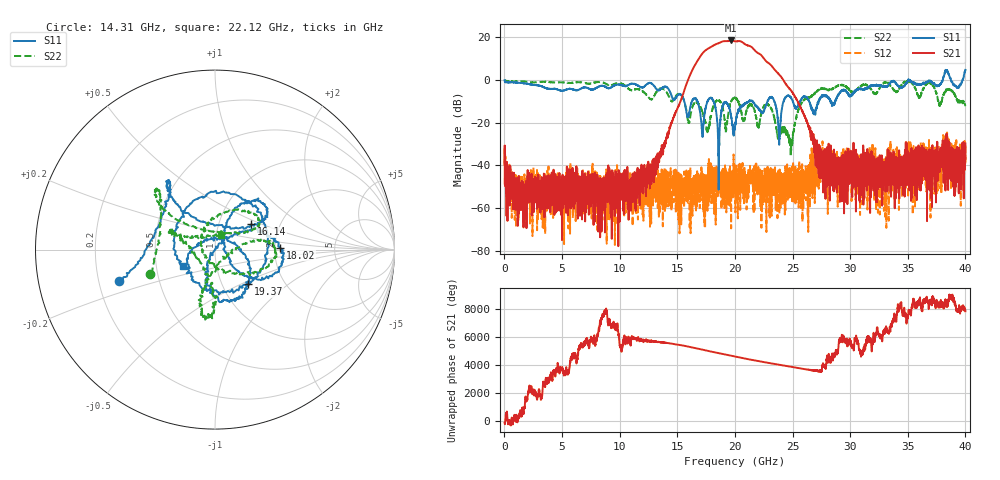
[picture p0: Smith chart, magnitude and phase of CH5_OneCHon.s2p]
!Keysight Technologies,N5245B,MY57181321,A.14.80.03
!Date: Thursday, March 28, 2024 17:39:08
!Correction: S11(C  2-Port  )
!S21(C  2-Port  )
!S12(C  2-Port  )
!S22(C  2-Port  )
!S2P File: Measurements: S11, S21, S12, S22:
# Hz S  RI  R 50
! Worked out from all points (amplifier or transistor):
!   4000 points, 10 MHz to 40 GHz, reference 50 ohm
!   highest |S21| = 18.5 dB at 19.63 GHz (marker M1)
!   |S21| within 3 dB of that: 17.92 GHz to 21.42 GHz (3.502 GHz wide, 17.8 % of centre)
!   unconditionally stable (mu >= 1): start of sweep to 35.03 GHz; 35.21 GHz to 38.03 GHz; 38.75 GHz to 39.75 GHz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
!   at 6.67 GHz: K = 7921.81, MAG = -45.0 dB, |S12| = -47.8 dB
!   at 20.01 GHz: K = 7.33, MAG = 18.8 dB, |S12| = -42.9 dB
!   at 40 GHz: K = -1587.78, MSG = 2.6 dB, |S12| = -34.9 dB
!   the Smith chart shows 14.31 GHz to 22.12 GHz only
!   S11 on the Smith chart (normalised r, x): 14.31 GHz: 0.28, -0.15; 16.14 GHz: 1.43, +0.43; 18.02 GHz: 2.13, +0.06; 19.37 GHz: 1.32, -0.55; 22.12 GHz: 0.68, -0.13
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1e7  0.982 -0.0438  -0.00761 -0.00725  0.0222 -0.0115  -0.9268 -0.0288
6.68e9  0.4256 0.4749  0.00112 0.00117  -0.00212 0.000551  0.8628 0.1787
1.334e10  -0.401 -0.4135  -0.0117 -0.0107  0.000694 0.00149  -0.5447 -0.2203
1.431e10  -0.5369 -0.1759  -0.0528 0.0478  -0.000634 -0.00254  -0.3623 -0.1358
1.614e10  0.2023 0.1413  -0.9274 -1.009  0.000359 -0.00182  0.1195 0.0945
1.698e10  0.0679 0.156  0.8558 3.417  0.00499 0.0021  0.0943 0.2168
1.745e10  0.1646 -0.1475  4.852 -0.935  0.00268 -0.0011  -0.0841 0.061
1.802e10  0.3616 0.0116  -2.486 -5.612  0.00151 0.00252  0.1388 -0.138
1.845e10  0.0928 0.0767  -6.982 0.9446  0.00262 -0.00119  0.3314 -0.0485
1.887e10  -0.0244 -0.1983  -1.553 7.699  -0.0032 0.00295  0.248 0.0493
1.937e10  0.1853 -0.1932  7.738 2.408  -0.00038 0.00183  -0.0146 -0.1246
1.963e10  0.1563 -0.0221  7.402 -3.993  -0.00108 -0.00274  -0.0825 -0.2795
2.001e10  -0.0723 0.0387  -0.1216 -8.047  -0.0063 0.00346  -0.0448 -0.3785
2.052e10  -0.0227 -0.227  -7.883 -1.011  -0.00154 0.00415  -0.0158 -0.1847
2.103e10  0.3001 0.0186  -0.9519 6.477  -0.00272 0.00336  -0.192 0.063
2.153e10  -0.0228 0.322  5.254 2.036  0.00427 -0.00261  -0.2384 0.0808
2.212e10  -0.1801 -0.0916  1.372 -3.843  -0.00224 -0.00465  0.0347 0.0832
2.268e10  0.2443 0.0213  -2.517 -1.189  -0.00175 -0.00351  0.2104 0.1667
2.332e10  -0.0327 0.3646  -0.856 1.709  -0.00218 -0.00269  0.1189 0.1092
2.667e10  0.1916 0.1024  0.0476 0.0253  -0.00472 -0.00766  0.3646 0.2084
3.334e10  0.6513 -0.4019  -0.00345 0.000405  -0.0107 0.00866  0.3027 -0.7605
4e10  0.2069 -1.717  -0.00901 -0.0314  -0.00124 0.0179  -0.0774 0.2442
